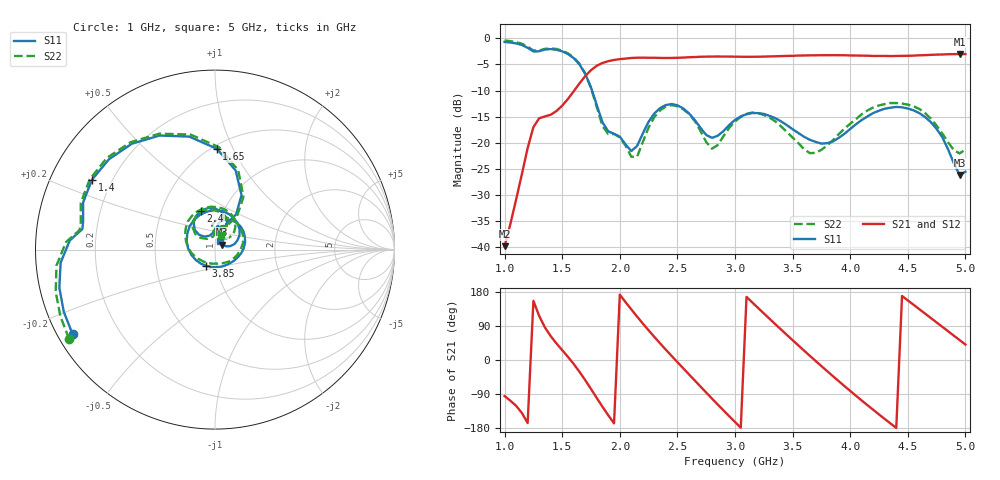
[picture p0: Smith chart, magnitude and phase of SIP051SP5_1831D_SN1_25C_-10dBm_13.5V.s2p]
# GHz  S  dB  R  50
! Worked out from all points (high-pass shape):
!   81 points, 1 GHz to 5 GHz, reference 50 ohm
!   highest |S21| = -3.03 dB at 4.95 GHz (marker M1); lowest = -39.8 dB at 1 GHz (marker M2)
!   |S21| within 3 dB of the highest: 1.755 GHz to end of sweep
!   lowest |S11| = -26.2 dB at 4.95 GHz (marker M3), VSWR 1.10, Z = 54.1 + j3.06 ohm
!   |S11| at or under -10 dB: 1.759 GHz to end of sweep
!   |S22| runs from -22.7 to -0.4 dB; largest |S21 - S12| = 0.0021
!   S11 on the Smith chart (normalised r, x): 1 GHz: 0.04, -0.27; 1.4 GHz: 0.13, +0.26; 1.65 GHz: 0.53, +0.87; 2.4 GHz: 0.78, +0.36; 3.85 GHz: 0.89, -0.16; 5 GHz: 1.05, +0.10
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1  -0.70 -149.3  -39.80 -95.2  -40.18 -94.1  -0.42 -148.5
1.25  -2.52 171.2  -17.01 156.2  -17.00 156.3  -2.35 171.9
1.4  -2.07 150.4  -14.64 63.1  -14.63 62.9  -1.94 150.7
1.65  -5.01 89.0  -8.64 -31.2  -8.64 -31.1  -4.87 87.7
1.7  -6.82 75.4  -7.24 -53.2  -7.25 -53.2  -6.75 73.6
1.85  -16.11 65.2  -4.72 -123.6  -4.71 -123.6  -16.83 64.6
2  -18.83 90.1  -3.99 172.4  -4.00 172.5  -18.97 88.7
2.2  -18.22 137.3  -3.72 96.1  -3.71 96.2  -19.85 140.6
2.35  -13.36 119.7  -3.76 43.8  -3.76 43.8  -13.80 125.3
2.4  -12.79 109.8  -3.77 27.1  -3.78 27.1  -13.05 114.7
2.55  -13.41 79.6  -3.69 -21.7  -3.69 -21.7  -13.59 81.2
2.75  -18.51 67.6  -3.52 -85.9  -3.51 -85.9  -19.87 65.4
3  -15.63 77.0  -3.52 -163.6  -3.52 -163.5  -15.94 89.8
3.15  -14.32 52.3  -3.54 151.9  -3.54 152.0  -14.22 60.3
3.35  -15.29 12.9  -3.45 94.5  -3.45 94.6  -15.90 13.4
3.7  -19.84 -67.9  -3.26 -2.6  -3.26 -2.5  -21.93 -101.9
3.85  -19.76 -118.3  -3.23 -42.6  -3.24 -42.6  -19.51 -150.8
4.1  -15.65 163.1  -3.32 -106.9  -3.32 -106.8  -14.55 152.8
4.35  -13.29 101.4  -3.41 -167.5  -3.41 -167.4  -12.40 105.1
4.7  -16.05 30.2  -3.17 110.8  -3.17 111.0  -15.39 48.2
4.95  -26.19 35.1  -3.03 52.5  -3.03 52.5  -22.05 58.4
5  -25.55 59.4  -3.03 40.9  -3.03 41.0  -21.31 69.0
